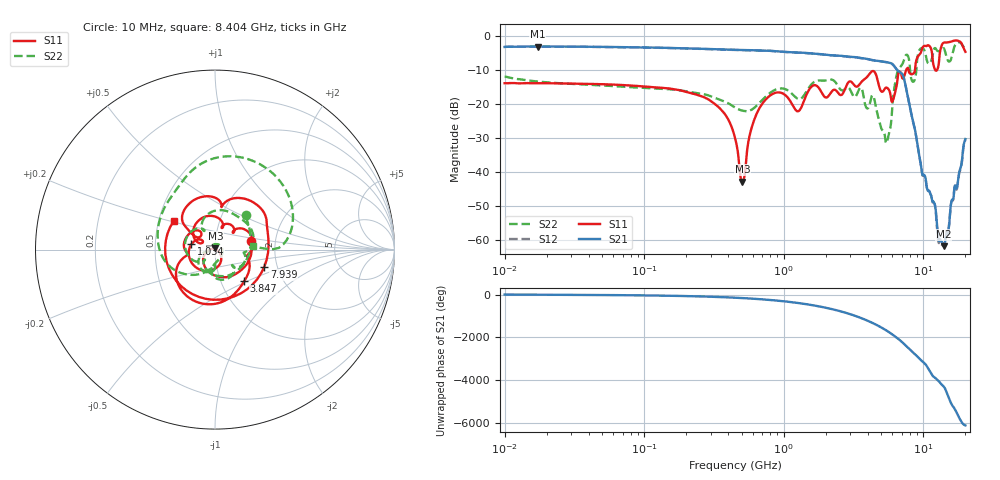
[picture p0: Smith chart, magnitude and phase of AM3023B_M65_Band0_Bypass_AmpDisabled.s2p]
!Agilent Technologies,E8364B,MY43040894,A.07.50.67
!Agilent E8364B: A.07.50.67
!Date: Tuesday, October 27, 2020 10:47:59
!Correction: S11(Full 2 Port(1,2))
!S21(Full 2 Port(1,2))
!S12(Full 2 Port(1,2))
!S22(Full 2 Port(1,2))
!S2P File: Measurements: S11, S21, S12, S22:Log Frequency Sweep
# Hz S  dB  R 50
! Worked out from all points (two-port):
!   3201 points, 10 MHz to 20 GHz, reference 50 ohm
!   highest |S21| = -2.99 dB at 17.23 MHz (marker M1); lowest = -61.7 dB at 14.04 GHz (marker M2)
!   |S21| within 3 dB of the highest: start of sweep to 2.906 GHz
!   lowest |S11| = -42.7 dB at 506 MHz (marker M3), VSWR 1.01, Z = 50.2 + j0.7 ohm
!   |S11| at or under -10 dB: start of sweep to 7.508 GHz; 7.835 GHz to 8.698 GHz (863.3 MHz wide, 10.4 % of centre); 12.2 GHz to 12.48 GHz (282.9 MHz wide, 2.29 % of centre)
!   |S22| runs from -31.4 to -1.7 dB; largest |S21 - S12| = 0.0075
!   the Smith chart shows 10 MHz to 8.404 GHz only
!   S11 on the Smith chart (normalised r, x): 10 MHz: 1.49, +0.15; 1.034 GHz: 0.77, +0.05; 3.847 GHz: 1.29, -0.48; 7.939 GHz: 1.71, -0.36; 8.404 GHz: 0.60, +0.21
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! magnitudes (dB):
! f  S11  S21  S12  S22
! 10 MHz  -13.8  -3.1  -3.1  -11.8
! 17.23 MHz  -13.8  -3.0  -3.0  -13.3
! 35.55 MHz  -13.9  -3.0  -3.1  -14.1
! 126.1 MHz  -15.0  -3.3  -3.4  -15.4
! 295.1 MHz  -18.8  -3.7  -3.8  -17.5
! 447.2 MHz  -29.8  -4.0  -4.0  -20.9
! 506 MHz  -42.7  -4.0  -4.1  -21.9
! 658.7 MHz  -21.6  -4.1  -4.1  -19.9
! 1.034 GHz  -17.4  -4.6  -4.6  -15.6
! 1.269 GHz  -22.0  -4.7  -4.8  -18.4
! 1.59 GHz  -14.7  -5.0  -5.1  -14.0
! 3.847 GHz  -12.4  -6.5  -6.6  -20.4
! 4.373 GHz  -10.2  -7.0  -7.1  -17.6
! 5.639 GHz  -15.6  -7.7  -7.7  -29.0
! 6.518 GHz  -12.9  -9.9  -9.9  -10.5
! 7.939 GHz  -10.7  -20.2  -20.2  -7.6
! 8.404 GHz  -11.0  -24.7  -24.8  -13.3
! 9.577 GHz  -4.8  -37.6  -37.6  -3.6
! 11.02 GHz  -2.8  -45.4  -45.6  -8.0
! 12.38 GHz  -10.1  -53.0  -53.9  -3.9
! 14.04 GHz  -1.8  -61.7  -61.3  -3.6
! 20 GHz  -4.5  -30.2  -30.5  -3.9
